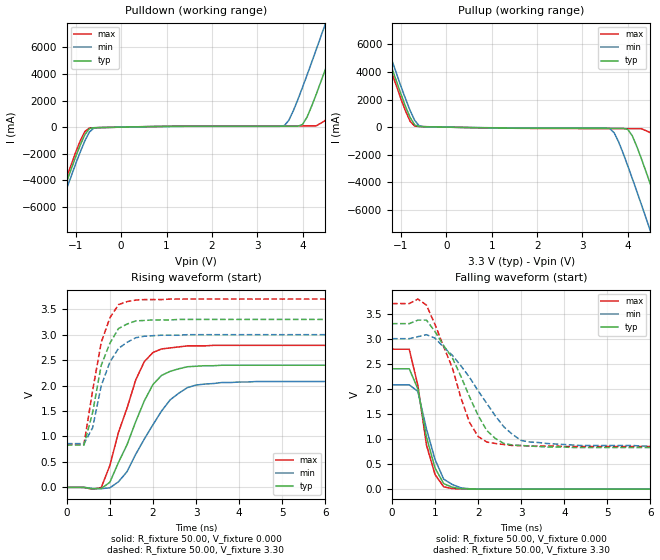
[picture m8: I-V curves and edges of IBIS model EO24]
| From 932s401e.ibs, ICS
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|   Model EO24
[Model]   EO24
Model_type   Output
Polarity   Non-Inverting
C_comp   2.50pF   2.00pF   3.00pF
[Temperature Range]   27.00   70.00   0.000
[Voltage Range]   3.30V   3.00V   3.70V
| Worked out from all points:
|   slope of the pulldown table from 0 to 0.495 V, typ, clamps not added: 15.1 ohm
|   slope of the pullup table from 0 to 0.495 V, typ, clamps not added: 17.1 ohm
|   rising waveform, R_fixture 50.00, V_fixture 0.000: 20-80 % time 743ps typ, 887ps min, 628ps max; typ from 0 V to 2.4 V
|   rising waveform, R_fixture 50.00, V_fixture 3.30: 20-80 % time 434ps typ, 455ps min, 408ps max; typ from 0.83 V to 3.3 V
|   falling waveform, R_fixture 50.00, V_fixture 0.000: 20-80 % time 364ps typ, 413ps min, 354ps max; typ from 2.4 V to 0 V
|   falling waveform, R_fixture 50.00, V_fixture 3.30: 20-80 % time 852ps typ, 1.06ns min, 695ps max; typ from 3.3 V to 0.83 V
[Pulldown]
| voltage   I(typ)   I(min)   I(max)
-3.3V     -24.56A    -25.26A    -24.25A
-1.7V     -8.82A     -9.35A     -8.5A
-1.5V     -6.89A     -7.42A     -6.56A
-900mV    -1.32A     -1.84A     -1.01A
-700mV    -110mA     -360mA     -63.12mA
3.6V      73.9mA     120mA      91.09mA
4V        200mA      3A         91.37mA
4.3V      2.45A      5.81A      92.16mA
4.5V      4.31A      7.73A      490mA
4.9V      8.15A      11.62A     3.97A
5.3V      12.06A     15.54A     7.82A
6.6V      24.92A     28.41A     20.63A
[Pullup]
| voltage   I(typ)   I(min)   I(max)
-3.3V     24.76A     25.29A     24.43A
-1.7V     9.02A      9.58A      8.68A
-1.5V     7.08A      7.65A      6.74A
-900mV    1.49A      2.04A      1.16A
-700mV    160mA      490mA      73.64mA
-500mV    33.31mA    32.07mA    36.48mA
3.6V      -85.86mA   -100mA     -110mA
4V        -160mA     -2.8A      -110mA
4.5V      -4.13A     -7.52A     -400mA
4.9V      -7.98A     -11.42A    -3.82A
5.3V      -11.89A    -15.35A    -7.67A
6.6V      -24.77A    -28.24A    -20.5A
[Ramp]
| variable   typ   min   max
dV/dt_r   1.44/0.68n   1.25/0.88n   1.67/0.56n
dV/dt_f   1.48/0.81n   1.28/1.04n   1.71/0.63n
R_load = 50.00
[Rising Waveform]
R_fixture = 50.00
V_fixture = 0.000
V_fixture_min = 0.000
V_fixture_max = 0.000
| time   V(typ)   V(min)   V(max)
0s        140uV      0V         190uV
800ps     -22.24mV   -24.99mV   -4.06mV
1ns       100mV      -8.92mV    430mV
1.4ns     840mV      310mV      1.56V
1.6ns     1.29V      650mV      2.11V
1.8ns     1.7V       950mV      2.47V
2.2ns     2.2V       1.5V       2.72V
2.8ns     2.37V      1.96V      2.78V
3.6ns     2.4V       2.06V      2.79V
10ns      2.4V       2.08V      2.79V
[Rising Waveform]
R_fixture = 50.00
V_fixture = 3.30
V_fixture_min = 3.00
V_fixture_max = 3.70
| time   V(typ)   V(min)   V(max)
0s        830mV      860mV      850mV
400ps     830mV      860mV      850mV
600ps     1.47V      1.17V      1.9V
800ps     2.4V       2V         2.85V
1ns       2.83V      2.46V      3.33V
1.2ns     3.12V      2.73V      3.59V
1.4ns     3.21V      2.85V      3.65V
1.6ns     3.27V      2.94V      3.68V
2.2ns     3.29V      2.99V      3.69V
10ns      3.3V       3V         3.7V
[Falling Waveform]
R_fixture = 50.00
V_fixture = 0.000
V_fixture_min = 0.000
V_fixture_max = 0.000
| time   V(typ)   V(min)   V(max)
0s        2.4V       2.08V      2.79V
400ps     2.4V       2.08V      2.79V
600ps     2V         1.95V      2.07V
800ps     1.04V      1.2V       880mV
1ns       420mV      590mV      290mV
1.2ns     110mV      200mV      47.02mV
1.4ns     38.27mV    92.75mV    11.81mV
1.6ns     8.29mV     26.57mV    3.5mV
2ns       2.44mV     3.2mV      2.07mV
10ns      -4.72uV    -3.13uV    3.4uV
[Falling Waveform]
R_fixture = 50.00
V_fixture = 3.30
V_fixture_min = 3.00
V_fixture_max = 3.70
| time   V(typ)   V(min)   V(max)
0s        3.3V       3V         3.7V
600ps     3.37V      3.04V      3.79V
800ps     3.37V      3.08V      3.67V
1.4ns     2.62V      2.67V      2.42V
1.8ns     1.84V      2.23V      1.33V
2ns       1.47V      1.96V      1.05V
2.2ns     1.17V      1.71V      940mV
2.6ns     910mV      1.24V      890mV
3.2ns     860mV      940mV      860mV
10ns      830mV      860mV      850mV
